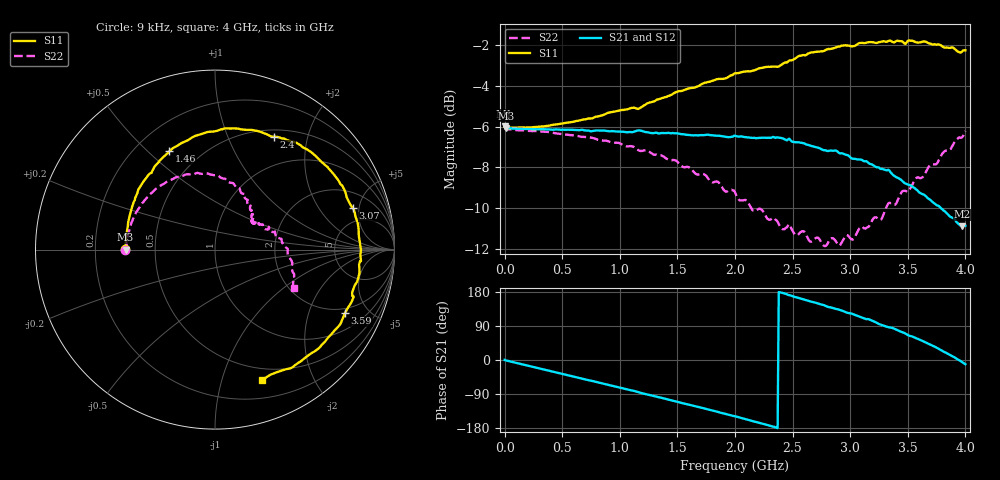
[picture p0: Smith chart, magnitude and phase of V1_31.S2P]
! ZVRE, 3.40
! symbol freq-unit parameter-type data-format keyword impedance-ohm
#  HZ  S  RI  R  50
! freq  reS11  imS11  reS21  imS21  reS12  imS12  reS22  imS22
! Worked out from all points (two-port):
!   401 points, 9 kHz to 4 GHz, reference 50 ohm
!   highest |S21| = -5.99 dB at 9 kHz (marker M1); lowest = -10.9 dB at 3.97 GHz (marker M2)
!   |S21| within 3 dB of the highest: start of sweep to 3.55 GHz
!   lowest |S11| = -6.1 dB at 10.01 MHz (marker M3), VSWR 2.98, Z = 16.8 + j0.018 ohm
!   |S11| at or under -10 dB: nowhere
!   |S22| runs from -11.9 to -6.0 dB; largest |S21 - S12| = 0.017
!   S11 on the Smith chart (normalised r, x): 9 kHz: 0.33, +0.00; 1.46 GHz: 0.34, +0.58; 2.4 GHz: 0.59, +1.49; 3.07 GHz: 3.35, +4.33; 3.59 GHz: 1.75, -3.53; 4 GHz: 0.38, -1.35
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9000  -0.4998 0.00109  0.5018 0.00123  0.5024 -0.00169  -0.5007 -0.000935
1.000898e7  -0.4979 0.000405  0.4963 -0.00883  0.4987 -0.00355  -0.4934 0.00819
3.300083e8  -0.4878 0.1173  0.4507 -0.2028  0.4553 -0.2003  -0.4543 0.1768
6.700075e8  -0.4603 0.2437  0.3231 -0.3717  0.3287 -0.3697  -0.3492 0.3191
1.010007e9  -0.3975 0.381  0.1367 -0.468  0.1405 -0.4702  -0.2078 0.4047
1.340006e9  -0.3004 0.5031  -0.0687 -0.4776  -0.0668 -0.4825  -0.0482 0.4236
1.460006e9  -0.2542 0.5475  -0.1447 -0.4615  -0.1416 -0.4647  0.00813 0.4153
1.740005e9  -0.1103 0.6336  -0.2968 -0.3749  -0.2958 -0.3775  0.1047 0.367
2.000004e9  0.0563 0.6757  -0.4063 -0.2493  -0.4036 -0.2508  0.1641 0.3046
2.400004e9  0.3295 0.6293  -0.4701 0.0168  -0.4687 0.0106  0.1947 0.2053
2.670003e9  0.5388 0.5406  -0.4015 0.2008  -0.4079 0.1922  0.2069 0.1612
2.850003e9  0.6487 0.4346  -0.3206 0.2977  -0.3314 0.2895  0.2153 0.1571
3.070002e9  0.7688 0.2301  -0.1802 0.3755  -0.1829 0.3812  0.2406 0.1414
3.190002e9  0.7976 0.1315  -0.0971 0.3929  -0.1039 0.3962  0.2601 0.1387
3.250002e9  0.8086 0.0282  -0.0336 0.3964  -0.0449 0.4013  0.2679 0.1272
3.340001e9  0.8133 -0.0631  0.0267 0.3903  0.0264 0.3938  0.3021 0.1222
3.530001e9  0.7661 -0.2792  0.1639 0.319  0.1625 0.3255  0.3509 0.0645
3.590001e9  0.7253 -0.3523  0.198 0.2861  0.1999 0.2924  0.3718 0.058
3.78e9  0.5682 -0.5576  0.2807 0.1488  0.2858 0.1486  0.4177 -0.0484
3.9e9  0.4133 -0.6633  0.2953 0.0415  0.296 0.0377  0.4373 -0.1308
3.97e9  0.2879 -0.7102  0.284 -0.026  0.2862 -0.0316  0.4361 -0.1798
4e9  0.2601 -0.727  0.2808 -0.055  0.28 -0.0568  0.4388 -0.2163
